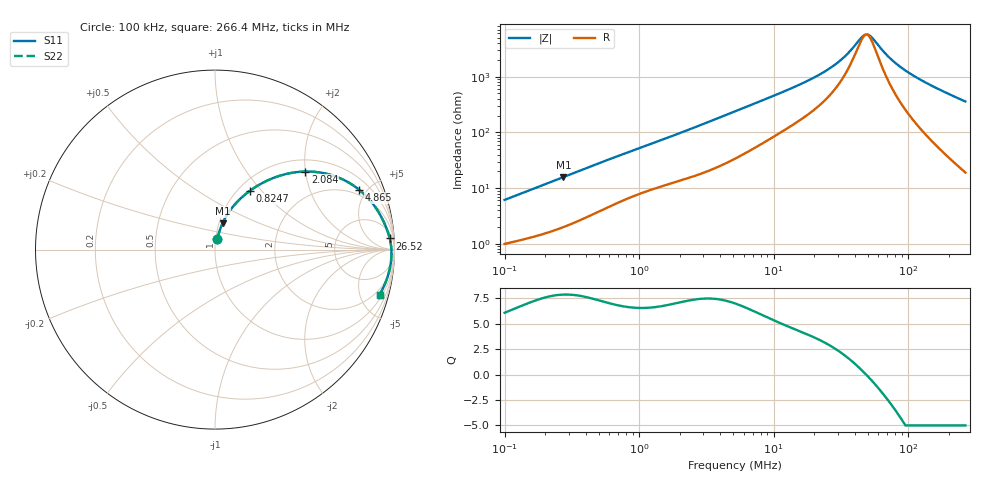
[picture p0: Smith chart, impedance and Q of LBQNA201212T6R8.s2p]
! LBQNA201212T6R8  S-PARAMETER MODEL  ( General Type )
! Model Generated by TAIYO YUDEN Corporation (http://www.ty-top.com)
! Version 1.0
! TAIYO YUDEN Control No. 191025NI43SB-FBB
! Copyright(c) 2019 TAIYO YUDEN CO.,LTD. All Rights Reserved.
! Product Description (link to TY-COMPAS)
! https://ds.yuden.co.jp/TYCOMPAS/or/detail?pn=LBQNA201212T6R8M&u=M
! Products Name : Inductors
! Characteristics :
!  Inductance : 6.8 uH , SRF(min) : 38 MHz , DC Resistance(max) : 0.611 Ohm
!  Rated Current : Saturation :250 mA , Temp Rise : 350 mA (20 degC)
!  Case Size : 2.0 x 1.25 / 0.079 x 0.049 [mm/inch] , Thickness : 1.25 / 0.049 [mm/inch]
!  (Conditions: Temperature = 25 degC , DC Bias Current/Voltage = 0A / 0V)
! External Node Assignments :
!  1  o---GGG---o  2
! GND o---------o GND
! Frequency Range : 0.1MHz  -  266.375554MHz  [ 402 STEP ]
# MHz S RI R 50
! Freq[MHz].  S11 Real  S11 Imag  S21 Real  S21 Imag  S12 Real  S12 Imag  S22 Real  S22 Imag
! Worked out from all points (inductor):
!   401 points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, 100 kHz to 266.4 MHz, reference 50 ohm
!   read as one part in series: L = 9.5 uH near 104 kHz
!   highest Q = 7.88 at 273.4 kHz (marker M1), where L = 9.15 uH
!   self-resonance near 48.77 MHz
!   S11 on the Smith chart (normalised r, x): 100 kHz: 1.02, +0.12; 824.7 kHz: 1.13, +0.87; 2.084 MHz: 1.28, +2.00; 4.865 MHz: 1.63, +4.47; 26.52 MHz: 11, +27; 266.4 MHz: 1.38, -7.17
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0.1  0.0134 0.0593  0.9866 -0.0593  0.9866 -0.0593  0.0134 0.0593
0.27337  0.0423 0.1475  0.9577 -0.1475  0.9577 -0.1475  0.0423 0.1475
0.374775  0.0663 0.1924  0.9337 -0.1924  0.9337 -0.1924  0.0663 0.1924
0.824745  0.1948 0.328  0.8052 -0.328  0.8052 -0.328  0.1948 0.328
1.404561  0.3518 0.4086  0.6482 -0.4086  0.6482 -0.4086  0.3518 0.4086
2.083605  0.5032 0.435  0.4968 -0.435  0.4968 -0.435  0.5032 0.435
3.030584  0.6531 0.4138  0.3469 -0.4138  0.3469 -0.4138  0.6531 0.4138
4.864699  0.8043 0.3326  0.1957 -0.3326  0.1957 -0.3326  0.8043 0.3326
5.26394  0.8233 0.3163  0.1767 -0.3163  0.1767 -0.3163  0.8233 0.3163
9.143143  0.9125 0.2068  0.0875 -0.2068  0.0875 -0.2068  0.9125 0.2068
19.34272  0.9631 0.0975  0.0369 -0.0975  0.0369 -0.0975  0.9631 0.0975
26.51779  0.9736 0.0619  0.0264 -0.0619  0.0264 -0.0619  0.9736 0.0619
32.94112  0.9783 0.0393  0.0217 -0.0393  0.0217 -0.0393  0.9783 0.0393
45.16044  0.9823 0.00768  0.0177 -0.00768  0.0177 -0.00768  0.9823 0.00768
48.86671  0.9829 -0.000197  0.0171 0.000197  0.0171 0.000197  0.9829 -0.000197
50.83239  0.9831 -0.00415  0.0169 0.00415  0.0169 0.00415  0.9831 -0.00415
53.93017  0.9833 -0.0101  0.0167 0.0101  0.0167 0.0101  0.9833 -0.0101
72.49162  0.9827 -0.0411  0.0173 0.0411  0.0173 0.0411  0.9827 -0.0411
90.05107  0.9805 -0.066  0.0195 0.066  0.0195 0.066  0.9805 -0.066
121.0445  0.974 -0.1048  0.026 0.1048  0.026 0.1048  0.974 -0.1048
179.5642  0.9556 -0.169  0.0444 0.169  0.0444 0.169  0.9556 -0.169
266.3756  0.9166 -0.2511  0.0834 0.2511  0.0834 0.2511  0.9166 -0.2511
